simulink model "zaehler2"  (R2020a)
settings: Solver=FixedStepDiscrete  StartTime=0.0  StopTime=Inf  FixedStep=1e-6  RelTol=1e-3  EnableMultiTasking=on

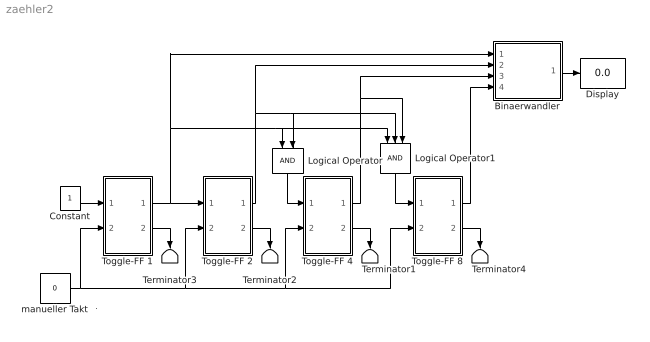
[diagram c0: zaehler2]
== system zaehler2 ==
  note: .
  Binaerwandler : Subsystem
  Constant : Constant
  Display : Display
  Logical Operator : Logic  AllPortsSameDT=off
  Logical Operator1 : Logic  Inputs=3  AllPortsSameDT=off
  Terminator{1..4} (4 alike) : Terminator
  Toggle-FF 1 : Subsystem
  Toggle-FF 2 : Subsystem
  Toggle-FF 4 : Subsystem
  Toggle-FF 8 : Subsystem
  manueller Takt : Constant  Value=0
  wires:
  manueller Takt/1 -> Toggle-FF 4/2(CLK), Toggle-FF 8/2(CLK), Toggle-FF 2/2(CLK), Toggle-FF 1/2(CLK)
  Binaerwandler/1(Out) -> Display/1
  Logical Operator1/1 -> Toggle-FF 8/1(T)
  Constant/1 -> Toggle-FF 1/1(T)
  Toggle-FF 1/2(!Q) -> Terminator3/1
  Toggle-FF 2/2(!Q) -> Terminator2/1
  Logical Operator/1 -> Toggle-FF 4/1(T)
  Toggle-FF 4/2(!Q) -> Terminator1/1
  Toggle-FF 8/2(!Q) -> Terminator4/1
  Toggle-FF 1/1(Q) -> Binaerwandler/1(In1), Logical Operator/1, Logical Operator1/1, Toggle-FF 2/1(T)
  Toggle-FF 2/1(Q) -> Binaerwandler/2(In2), Logical Operator/2, Logical Operator1/2
  Toggle-FF 4/1(Q) -> Binaerwandler/3(In4), Logical Operator1/3
  Toggle-FF 8/1(Q) -> Binaerwandler/4(In8)

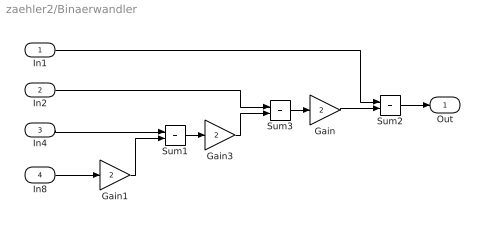
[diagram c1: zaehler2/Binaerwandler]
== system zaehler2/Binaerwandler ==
  In1 : Inport
  In2 : Inport  Port=2
  In4 : Inport  Port=3
  In8 : Inport  Port=4
  Gain : Gain  Gain=2  SaturateOnIntegerOverflow=on
  Gain1 : Gain  Gain=2  SaturateOnIntegerOverflow=on
  Gain3 : Gain  Gain=2  SaturateOnIntegerOverflow=on
  Sum1 : Sum  SaturateOnIntegerOverflow=on
  Sum2 : Sum  SaturateOnIntegerOverflow=on
  Sum3 : Sum  SaturateOnIntegerOverflow=on
  Out : Outport
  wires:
  Gain/1 -> Sum2/2
  In1/1 -> Sum2/1
  Sum2/1 -> Out/1
  Sum3/1 -> Gain/1
  In2/1 -> Sum3/1
  Gain3/1 -> Sum3/2
  Sum1/1 -> Gain3/1
  In4/1 -> Sum1/1
  Gain1/1 -> Sum1/2
  In8/1 -> Gain1/1

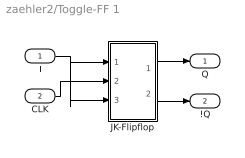
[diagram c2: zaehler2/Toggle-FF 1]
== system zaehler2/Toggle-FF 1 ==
  T : Inport
  CLK : Inport  Port=2
  JK-Flipflop : Subsystem  mask(JKFlipFlop){initial_condition=0}
      mask prompts: initial_condition "Initial condition (state of Q):"
      mask help: J-K Flip-Flop Block (Negative Edge Triggered)
  Q : Outport
  !Q : Outport  Port=2
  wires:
  JK-Flipflop/2(!Q) -> !Q/1
  CLK/1 -> JK-Flipflop/2(CLK)
  JK-Flipflop/1(Q) -> Q/1
  T/1 -> JK-Flipflop/1(J), JK-Flipflop/3(K)

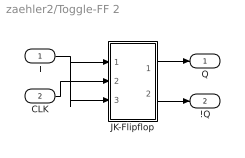
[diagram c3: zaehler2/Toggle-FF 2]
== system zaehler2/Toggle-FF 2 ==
  T : Inport
  CLK : Inport  Port=2
  JK-Flipflop : Subsystem  mask(JKFlipFlop){initial_condition=0}
      mask prompts: initial_condition "Initial condition (state of Q):"
      mask help: J-K Flip-Flop Block (Negative Edge Triggered)
  Q : Outport
  !Q : Outport  Port=2
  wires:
  JK-Flipflop/2(!Q) -> !Q/1
  CLK/1 -> JK-Flipflop/2(CLK)
  JK-Flipflop/1(Q) -> Q/1
  T/1 -> JK-Flipflop/1(J), JK-Flipflop/3(K)

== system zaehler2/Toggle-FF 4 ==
  T : Inport
  CLK : Inport  Port=2
  JK-Flipflop : Subsystem  mask(JKFlipFlop){initial_condition=0}
      mask prompts: initial_condition "Initial condition (state of Q):"
      mask help: J-K Flip-Flop Block (Negative Edge Triggered)
  Q : Outport
  !Q : Outport  Port=2
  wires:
  JK-Flipflop/2(!Q) -> !Q/1
  CLK/1 -> JK-Flipflop/2(CLK)
  JK-Flipflop/1(Q) -> Q/1
  T/1 -> JK-Flipflop/1(J), JK-Flipflop/3(K)

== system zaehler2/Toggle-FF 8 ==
  T : Inport
  CLK : Inport  Port=2
  JK-Flipflop : Subsystem  mask(JKFlipFlop){initial_condition=0}
      mask prompts: initial_condition "Initial condition (state of Q):"
      mask help: J-K Flip-Flop Block (Negative Edge Triggered)
  Q : Outport
  !Q : Outport  Port=2
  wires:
  JK-Flipflop/2(!Q) -> !Q/1
  CLK/1 -> JK-Flipflop/2(CLK)
  JK-Flipflop/1(Q) -> Q/1
  T/1 -> JK-Flipflop/1(J), JK-Flipflop/3(K)

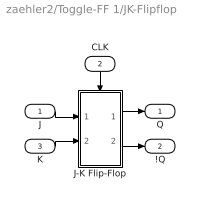
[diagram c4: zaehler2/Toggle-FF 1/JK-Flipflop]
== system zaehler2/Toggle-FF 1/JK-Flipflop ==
  J : Inport
  CLK : Inport  Port=2
  K : Inport  Port=3
  J-K Flip-Flop : Subsystem  TreatAsAtomicUnit=on
  Q : Outport
  !Q : Outport  Port=2
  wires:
  CLK/1 -> J-K Flip-Flop/Trigger
  J-K Flip-Flop/1(Q) -> Q/1
  J/1 -> J-K Flip-Flop/1(J)
  K/1 -> J-K Flip-Flop/2(K)
  J-K Flip-Flop/2(!Q) -> !Q/1

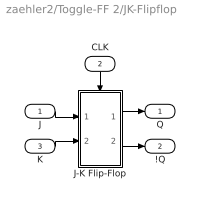
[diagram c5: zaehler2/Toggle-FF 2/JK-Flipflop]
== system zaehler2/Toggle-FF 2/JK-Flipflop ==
  J : Inport
  CLK : Inport  Port=2
  K : Inport  Port=3
  J-K Flip-Flop : Subsystem  TreatAsAtomicUnit=on
  Q : Outport
  !Q : Outport  Port=2
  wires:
  CLK/1 -> J-K Flip-Flop/Trigger
  J-K Flip-Flop/1(Q) -> Q/1
  J/1 -> J-K Flip-Flop/1(J)
  K/1 -> J-K Flip-Flop/2(K)
  J-K Flip-Flop/2(!Q) -> !Q/1

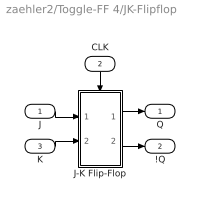
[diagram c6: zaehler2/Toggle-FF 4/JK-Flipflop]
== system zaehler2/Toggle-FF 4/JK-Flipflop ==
  J : Inport
  CLK : Inport  Port=2
  K : Inport  Port=3
  J-K Flip-Flop : Subsystem  TreatAsAtomicUnit=on
  Q : Outport
  !Q : Outport  Port=2
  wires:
  CLK/1 -> J-K Flip-Flop/Trigger
  J-K Flip-Flop/1(Q) -> Q/1
  J/1 -> J-K Flip-Flop/1(J)
  K/1 -> J-K Flip-Flop/2(K)
  J-K Flip-Flop/2(!Q) -> !Q/1

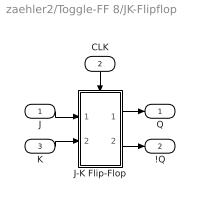
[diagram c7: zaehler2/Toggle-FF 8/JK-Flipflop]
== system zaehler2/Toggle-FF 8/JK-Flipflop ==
  J : Inport
  CLK : Inport  Port=2
  K : Inport  Port=3
  J-K Flip-Flop : Subsystem  TreatAsAtomicUnit=on
  Q : Outport
  !Q : Outport  Port=2
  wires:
  CLK/1 -> J-K Flip-Flop/Trigger
  J-K Flip-Flop/1(Q) -> Q/1
  J/1 -> J-K Flip-Flop/1(J)
  K/1 -> J-K Flip-Flop/2(K)
  J-K Flip-Flop/2(!Q) -> !Q/1

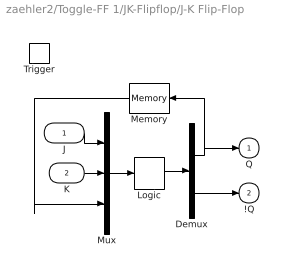
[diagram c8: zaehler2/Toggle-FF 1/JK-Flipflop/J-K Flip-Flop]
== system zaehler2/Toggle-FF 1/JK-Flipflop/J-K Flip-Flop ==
  J : Inport
  K : Inport  Port=2
  Trigger : TriggerPort  TriggerType=falling  VariantControl=Variant
  Demux : Demux  Outputs=2
  Logic : CombinatorialLogic  TruthTable=[0 1; 1 0; 0 1; 0 1; 1 0; 1 0; 1 0; 0 1]
  Memory : Memory  InitialCondition=initial_condition  InheritSampleTime=on
  Mux : Mux  Inputs=3
  Q : Outport  InitialOutput=initial_condition
  !Q : Outport  Port=2  InitialOutput=~initial_condition
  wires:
  Mux/1 -> Logic/1
  Logic/1 -> Demux/1
  Demux/2 -> !Q/1
  Demux/1 -> Memory/1, Q/1
  J/1 -> Mux/1
  K/1 -> Mux/2
  Memory/1 -> Mux/3

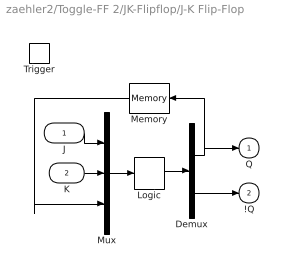
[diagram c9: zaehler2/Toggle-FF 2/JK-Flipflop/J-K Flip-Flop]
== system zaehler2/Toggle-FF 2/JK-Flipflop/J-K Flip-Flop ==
  J : Inport
  K : Inport  Port=2
  Trigger : TriggerPort  TriggerType=falling  VariantControl=Variant
  Demux : Demux  Outputs=2
  Logic : CombinatorialLogic  TruthTable=[0 1; 1 0; 0 1; 0 1; 1 0; 1 0; 1 0; 0 1]
  Memory : Memory  InitialCondition=initial_condition  InheritSampleTime=on
  Mux : Mux  Inputs=3
  Q : Outport  InitialOutput=initial_condition
  !Q : Outport  Port=2  InitialOutput=~initial_condition
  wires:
  Mux/1 -> Logic/1
  Logic/1 -> Demux/1
  Demux/2 -> !Q/1
  Demux/1 -> Memory/1, Q/1
  J/1 -> Mux/1
  K/1 -> Mux/2
  Memory/1 -> Mux/3

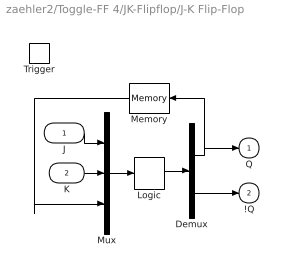
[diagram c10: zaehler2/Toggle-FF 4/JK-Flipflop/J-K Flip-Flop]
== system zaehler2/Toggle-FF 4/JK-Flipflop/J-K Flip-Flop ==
  J : Inport
  K : Inport  Port=2
  Trigger : TriggerPort  TriggerType=falling  VariantControl=Variant
  Demux : Demux  Outputs=2
  Logic : CombinatorialLogic  TruthTable=[0 1; 1 0; 0 1; 0 1; 1 0; 1 0; 1 0; 0 1]
  Memory : Memory  InitialCondition=initial_condition  InheritSampleTime=on
  Mux : Mux  Inputs=3
  Q : Outport  InitialOutput=initial_condition
  !Q : Outport  Port=2  InitialOutput=~initial_condition
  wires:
  Mux/1 -> Logic/1
  Logic/1 -> Demux/1
  Demux/2 -> !Q/1
  Demux/1 -> Memory/1, Q/1
  J/1 -> Mux/1
  K/1 -> Mux/2
  Memory/1 -> Mux/3

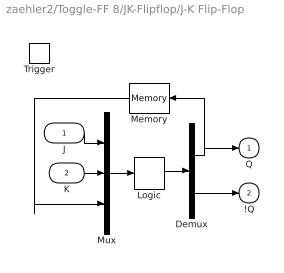
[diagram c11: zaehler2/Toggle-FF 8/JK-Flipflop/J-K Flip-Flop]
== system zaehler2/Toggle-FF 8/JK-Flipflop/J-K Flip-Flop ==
  J : Inport
  K : Inport  Port=2
  Trigger : TriggerPort  TriggerType=falling  VariantControl=Variant
  Demux : Demux  Outputs=2
  Logic : CombinatorialLogic  TruthTable=[0 1; 1 0; 0 1; 0 1; 1 0; 1 0; 1 0; 0 1]
  Memory : Memory  InitialCondition=initial_condition  InheritSampleTime=on
  Mux : Mux  Inputs=3
  Q : Outport  InitialOutput=initial_condition
  !Q : Outport  Port=2  InitialOutput=~initial_condition
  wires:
  Mux/1 -> Logic/1
  Logic/1 -> Demux/1
  Demux/2 -> !Q/1
  Demux/1 -> Memory/1, Q/1
  J/1 -> Mux/1
  K/1 -> Mux/2
  Memory/1 -> Mux/3
